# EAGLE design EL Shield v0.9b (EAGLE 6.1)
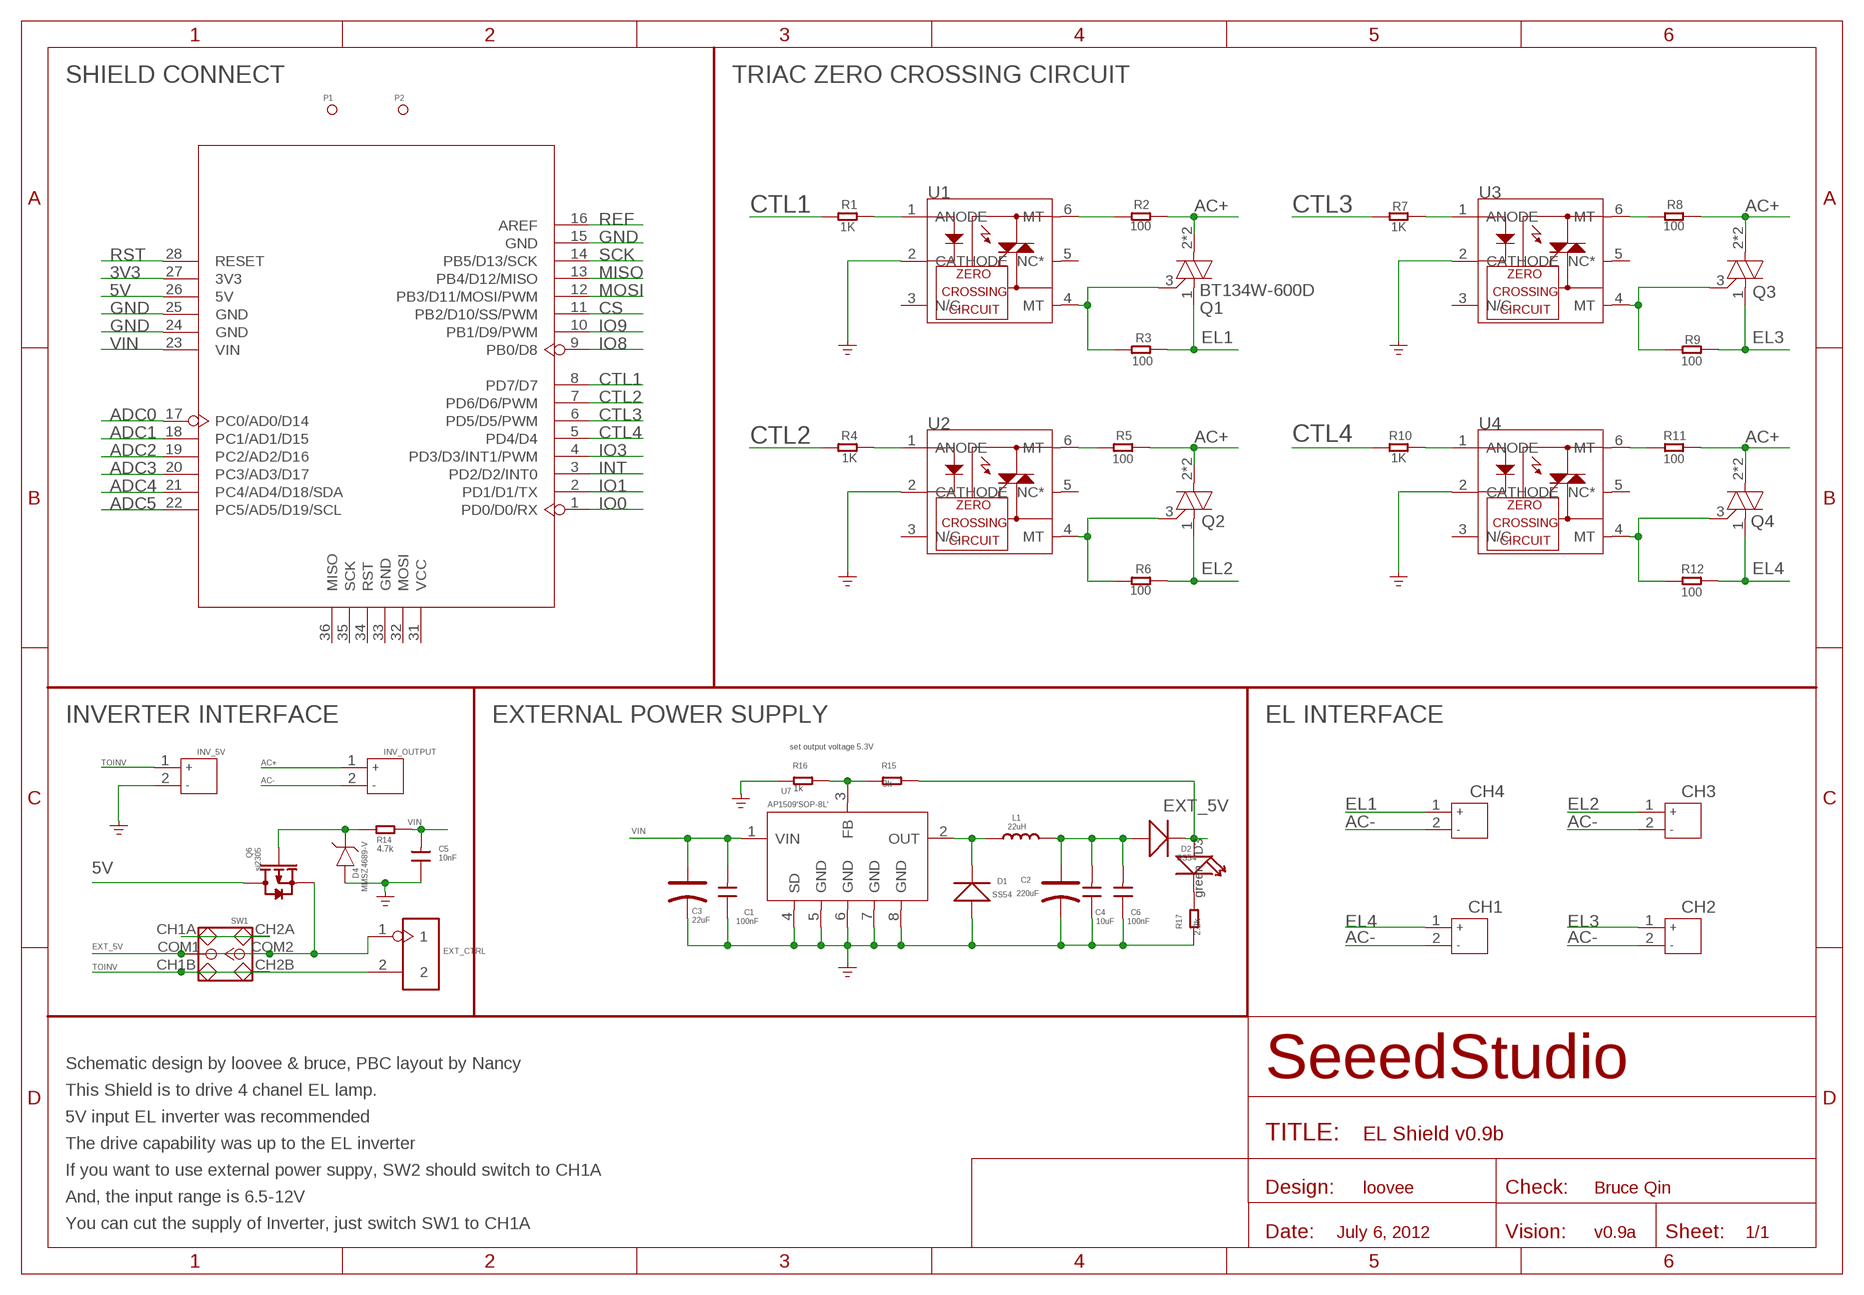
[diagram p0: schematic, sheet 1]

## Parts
C1  100nF  C-0603  [0603]
C2  220uF  CAP-AVX-B  [AVX-B]
C3  22uF  CAP-AVX-A  [AVX-A]
C4  10uF  C-0603  [0603]
C5  10nF  C-0603  [0603]
C6  100nF  C-0603  [0603]
CH1  JACK-JST-2P-PW'SMD'  [JST-SMD-2.0]
CH2  JACK-JST-2P-PW'SMD'  [JST-SMD-2.0]
CH3  JACK-JST-2P-PW'SMD'  [JST-SMD-2.0]
CH4  JACK-JST-2P-PW'SMD'  [JST-SMD-2.0]
D1  SS54  D'MBRS240LT3'  [SMB]
D2  SS54  D'MBRS240LT3'  [SMB]
D3  green  LED'0603'  [LED-0603]
D4  MMSZ4689-V  D-VOL'MMSZ4681'  [SOD123-2.7X1.6]
EXT_CTRL  HEADER-2P-65/35MIL  [2P-2.54-65/35MIL]
INV_5V  JACK-JST-2P-PW'2.0'  [JST-2.0]
INV_OUTPUT  JACK-JST-2P-PW'2.0'  [JST-2.0]
L1  22uH  L'2218'  [2218]
P1  PAD-MARK  [ROUND-MARK-1.0]
P2  PAD-MARK  [ROUND-MARK-1.0]
Q1  BT134W-600D  TRIAC'BT134W-600D'  [SOT-223]
Q2  TRIAC'BT134W-600D'  [SOT-223]
Q3  TRIAC'BT134W-600D'  [SOT-223]
Q4  TRIAC'BT134W-600D'  [SOT-223]
Q6  si2305  MOSFET-P'SI2323CDS/SI2305DS<BR>'  [SOT23]
R1  1K  R-0603  [R0603]
R2  100  R-0805  [R0805]
R3  100  R-0805  [R0805]
R4  1K  R-0603  [R0603]
R5  100  R-0805  [R0805]
R6  100  R-0805  [R0805]
R7  1K  R-0603  [R0603]
R8  100  R-0805  [R0805]
R9  100  R-0805  [R0805]
R10  1K  R-0603  [R0603]
R11  100  R-0805  [R0805]
R12  100  R-0805  [R0805]
R14  4.7k  R-0603  [R0603]
R15  3k  R-0603  [R0603]
R16  1k  R-0603  [R0603]
R17  2.2k  R-0603  [R0603]
SW1  SWITCH-2CH-6P  [6P-2CH-2.54-7.6X3.0]
U1  MOC3063MS  [SM6]
U2  MOC3063MS  [SM6]
U3  MOC3063MS  [SM6]
U4  MOC3063MS  [SM6]
U5  ARDUINO  [ARDUINO]
U7  AP1509'SOP-8L'  [SOP8-6.0-4.9X3.9]

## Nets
3V3: U5.27(3V3)
5V: Q6.3(D) U5.26(5V)
AC+: INV_OUTPUT.1 Q1.2(T2) Q1.TER(T2) Q2.2(T2) Q2.TER(T2) Q3.2(T2) Q3.TER(T2) Q4.2(T2) Q4.TER(T2) R2.2 R5.2 R8.2 R11.2
AC-: CH1.2 CH2.2 CH3.2 CH4.2 INV_OUTPUT.2
ADC0: U5.17(PC0/AD0/D14)
ADC1: U5.18(PC1/AD1/D15)
ADC2: U5.19(PC2/AD2/D16)
ADC3: U5.20(PC3/AD3/D17)
ADC4: U5.21(PC4/AD4/D18/SDA)
ADC5: U5.22(PC5/AD5/D19/SCL)
CS: U5.11(PB2/D10/SS/PWM)
CTL1: R1.2 U5.8(PD7/D7)
CTL2: R4.2 U5.7(PD6/D6/PWM)
CTL3: R7.2 U5.6(PD5/D5/PWM)
CTL4: R10.2 U5.5(PD4/D4)
EL1: CH4.1 Q1.1(T1) R3.2
EL2: CH3.1 Q2.1(T1) R6.2
EL3: CH2.1 Q3.1(T1) R9.2
EL4: CH1.1 Q4.1(T1) R12.2
EXT_5V: D2.- D3.+ EXT_CTRL.1 Q6.2(S) R15.1 SW1.COM1 SW1.COM2
GND: C1.1 C2.- C3.- C4.1 C5.1 C6.1 D1.+ D4.1 INV_5V.2 R16.2 R17.2 U1.2(CATHODE) U2.2(CATHODE) U3.2(CATHODE) U4.2(CATHODE) U5.15(GND) U5.24(GND) U5.25(GND) U7.4(SD) U7.5(GND) U7.6(GND) U7.7(GND) U7.8(GND)
INT: U5.3(PD2/D2/INT0)
IO0: U5.1(PD0/D0/RX)
IO1: U5.2(PD1/D1/TX)
IO3: U5.4(PD3/D3/INT1/PWM)
IO8: U5.9(PB0/D8)
IO9: U5.10(PB1/D9/PWM)
MISO: U5.13(PB4/D12/MISO)
MOSI: U5.12(PB3/D11/MOSI/PWM)
N$1: SW1.CH1A SW1.CH2A
N$2: R4.1 U2.1(ANODE)
N$3: R5.1 U2.6(MT)
N$4: Q2.3(G) R6.1 U2.4(MT)
N$5: R15.2 R16.1 U7.3(FB)
N$6: R7.1 U3.1(ANODE)
N$7: R8.1 U3.6(MT)
N$8: Q3.3(G) R9.1 U3.4(MT)
N$9: D4.2 Q6.1(G) R14.1
N$10: D1.- L1.P$1 U7.2(OUT)
N$11: R1.1 U1.1(ANODE)
N$12: R2.1 U1.6(MT)
N$13: R10.1 U4.1(ANODE)
N$14: Q1.3(G) R3.1 U1.4(MT)
N$15: R11.1 U4.6(MT)
N$16: Q4.3(G) R12.1 U4.4(MT)
N$17: D3.- R17.1
N$18: C2.+ C4.2 C6.2 D2.+ L1.P$2
REF: U5.16(AREF)
RST: U5.28(RESET)
SCK: U5.14(PB5/D13/SCK)
TOINV: EXT_CTRL.2 INV_5V.1 SW1.CH1B SW1.CH2B
VIN: C1.2 C3.+ C5.2 R14.2 U5.23(VIN) U7.1(VIN)
Unconnected: U1.3(N/C) U1.5(NC*) U2.3(N/C) U2.5(NC*) U3.3(N/C) U3.5(NC*) U4.3(N/C) U4.5(NC*) U5.31(VCC) U5.32(MOSI) U5.33(GND) U5.34(RST) U5.35(SCK) U5.36(MISO)

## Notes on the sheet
- SHIELD CONNECT | TRIAC ZERO CROSSING CIRCUIT
- INVERTER INTERFACE | EXTERNAL POWER SUPPLY | EL INTERFACE
- set output voltage 5.3V
- Schematic design by loovee & bruce, PBC layout by Nancy
- This Shield is to drive 4 chanel EL lamp.
- 5V input EL inverter was recommended
- The drive capability was up to the EL inverter
- If you want to use external power suppy, SW2 should switch to CH1A
- loovee | Bruce Qin
- And, the input range is 6.5-12V
- You can cut the supply of Inverter, just switch SW1 to CH1A
- July 6, 2012 | v0.9a

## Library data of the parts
C1 C4-C6 = Discrete:C*: Ceramic Capacitors
C2 C3 = Discrete:CAP*: Electrolytic Capacitors,Tantalum Capacitors and Super Capacitors
CH1-CH4 INV_5V INV_OUTPUT = Connector:JACK-JST-2P-PW
D1 D2 = Discrete:D*
D3 = Discrete:LED*
D4 = template:D-VOL
EXT_CTRL = Connector:HEADER-2P
L1 = Discrete:L*
P1 P2 = Discrete:PAD-MARK; PARTNO: DNP
Q1-Q4 = template:TRIAC: Triac
Q6 = Discrete:MOSFET-P
R1-R12 R14-R17 = Discrete:R*
SW1 = Discrete:SWITCH-2CH-6P
U1-U4 = template:MOC3063*M: 6-Pin DIP Zero-Cross Phototriac Driver Optocoupler(600 Volt Peak)
U5 = moudle:ARDUINO
U7 = IC:AP1509: 150KHz,2A PWM Buck DC/DC Converter

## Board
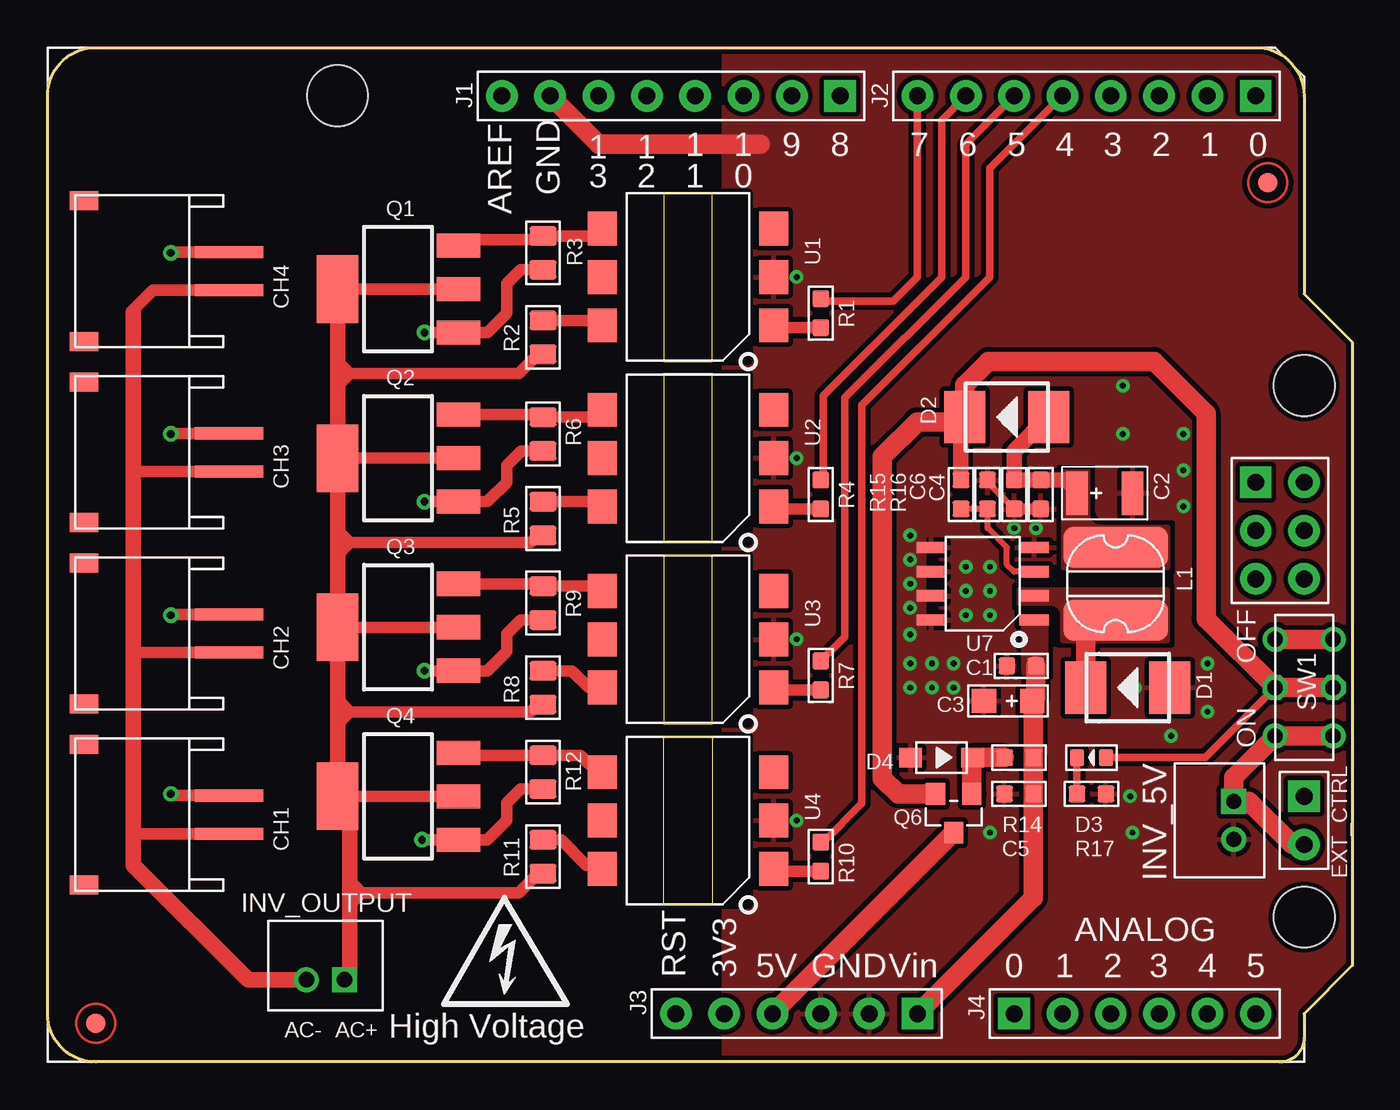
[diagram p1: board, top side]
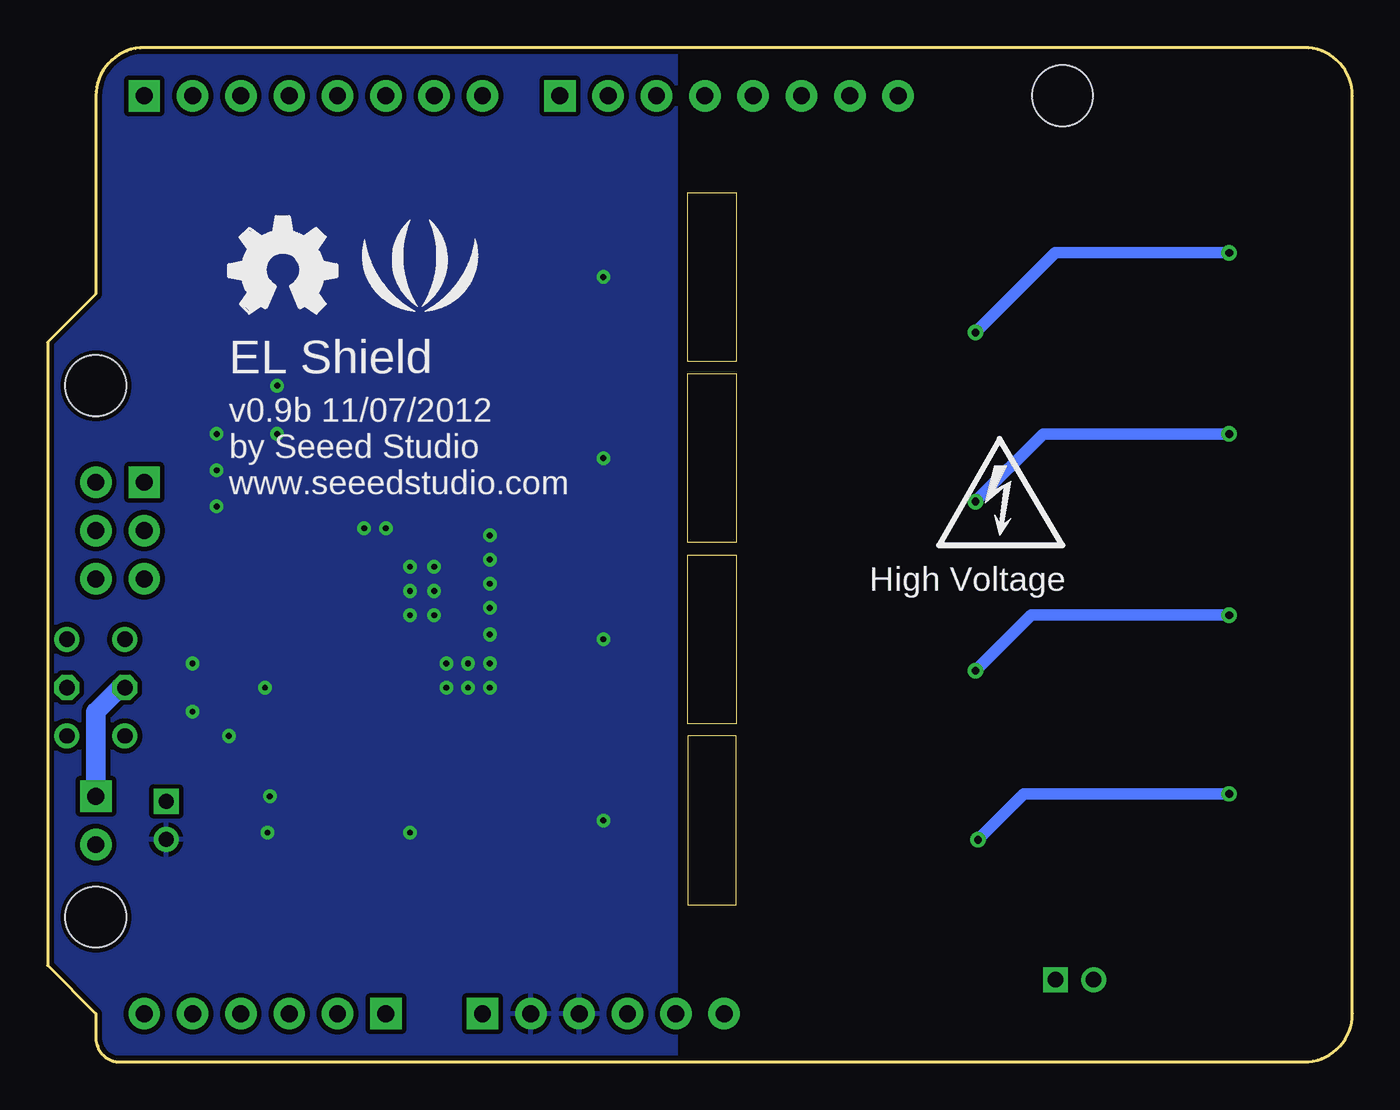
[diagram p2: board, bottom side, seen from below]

Size 68.58 x 53.34 mm. Coordinates in mm from the lower left corner, seen from the top.
Outline: 32.38,17.14 34.92,17.14 34.92,8.25 32.38,8.25 32.38,17.14
Outline: 32.38,17.78 34.92,17.78 34.92,26.67 32.38,26.67 32.38,17.78
Outline: 32.38,27.3 34.92,27.3 34.92,36.19 32.38,36.19 32.38,27.3
Outline: 32.38,36.83 34.92,36.83 34.92,45.72 32.38,45.72 32.38,36.83
Outline: 66.04,2.54 66.04,1.27 arc-90 64.77,0 2.54,0 arc-90 0,2.54 0,50.8 arc-90 2.54,53.34 63.5,53.34 arc-90 66.04,50.8 66.04,40.39 68.58,37.85 68.58,5.08 66.04,2.54
Copper layers (1*16): Top 0.035mm / dielectric 1.5mm / Bottom 0.035mm
Design rules: minimum track width 10mil, minimum drill 12mil, track to track 8mil, track to pad 8mil, pad to pad 8mil, via to via 8mil, smd to smd 0mil, copper to edge 10mil, drill to drill 8mil, minimum pad ring 10mil, minimum via ring 8mil, stop-mask expansion 4mil, vias tented up to drill 100mil, thermal gap 10mil
tRestrict: area 53.2,25.3 to 58.9,25.5; area 46.2,23.7 to 46.6,24; area 46.2,25 to 46.6,25.3; area 46.2,26.3 to 46.6,26.5

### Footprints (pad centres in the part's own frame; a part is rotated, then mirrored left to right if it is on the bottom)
0603 = smd 0.889 x 0.889: 1 -0.762,0; 2 0.762,0
AVX-B = smd 1.143 x 2.286: + -1.46,0; - 1.46,0
AVX-A = smd 1.27 x 1.27: + -1.27,0; - 1.27,0
JST-SMD-2.0 = smd 0.635 x 3.6: 1 -1,5.08; 2 1,5.08 | smd 1 x 1.5: P$1 -3.7,-2.54; P$2 3.7,-2.54
SMB = smd 2.159 x 2.743: + -2.21,0.254; - 2.21,0.254
LED-0603 = smd 0.762 x 0.889: + -0.762,0; - 0.762,0
SOD123-2.7X1.6 = smd 1.2 x 1.02: 1 -1.635,0; 2 1.635,0
2P-2.54-65/35MIL = drill 0.889 pad 1.651 square: 1 0,1.27 | drill 0.889 pad 1.651: 2 0,-1.27
JST-2.0 = drill 0.8 pad 1.3 square: 1 -1,0.75 | drill 0.8 pad 1.3: 2 1,0.75
2218 = smd 2.15 x 5.5: P$1 -1.925,0; P$2 1.925,0
ROUND-MARK-1.0 = smd 1.016 x 1.016: P$1 0,0
SOT-223 = smd 1.27 x 2.286: 1 -2.286,-3.175; 2 0,-3.175; 3 2.286,-3.175 | smd 3.556 x 2.159: TER 0,3.175
SOT23 = smd 1.016 x 1.143: 1 -0.95,-1.016; 2 0.95,-1.016; 3 0,1.016
R0603 = smd 0.889 x 0.889: 1 -0.762,0; 2 0.762,0
R0805 = smd 1.016 x 1.397: 1 -0.889,0; 2 0.889,0
6P-2CH-2.54-7.6X3.0 = drill 0.813 pad 1.27: CH1A -1.524,2.54; CH1B -1.524,-2.54; CH2A 1.524,2.54; CH2B 1.524,-2.54 | drill 0.813 pad 1.27 octagon: COM1 -1.524,0; COM2 1.524,0
SM6 = smd 1.78 x 1.52: 1 -2.54,-4.505; 2 0,-4.505; 3 2.54,-4.505; 4 2.54,4.505; 5 0,4.505; 6 -2.54,4.505
ARDUINO = drill 0.889 pad 1.651 square: 1 63.5,50.8; 9 41.656,50.8; 17 50.8,2.54; 23 45.72,2.54; 36 63.5,30.48 | drill 0.889 pad 1.651: 2 60.96,50.8; 3 58.42,50.8; 4 55.88,50.8; 5 53.34,50.8; 6 50.8,50.8; 7 48.26,50.8; 8 45.72,50.8; 10 39.116,50.8; 11 36.576,50.8; 12 34.036,50.8; 13 31.496,50.8; 14 28.956,50.8; 15 26.416,50.8; 16 23.876,50.8; 18 53.34,2.54; 19 55.88,2.54; 20 58.42,2.54; 21 60.96,2.54; 22 63.5,2.54; 24 43.18,2.54; 25 40.64,2.54; 26 38.1,2.54; 27 35.56,2.54; 28 33.02,2.54; 31 66.04,30.48; 32 66.04,27.94; 33 66.04,25.4; 34 63.5,25.4; 35 63.5,27.94 | hole 3.2: 15.24,50.8; 66.04,35.56; 66.04,7.62
SOP8-6.0-4.9X3.9 = smd 0.6 x 1.55: 1 -1.905,-2.7; 2 -0.635,-2.7; 3 0.635,-2.7; 4 1.905,-2.7; 5 1.905,2.7; 6 0.635,2.7; 7 -0.635,2.7; 8 -1.905,2.7

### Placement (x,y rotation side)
C1  51.18,20.83 0 top
C2  55.56,29.91 0 top
C3  50.48,18.99 180 top
C4  52.2,29.84 90 top
C5  51.05,14.1 0 top
C6  50.8,29.84 90 top
CH1  4.44,13 270 top
CH2  4.44,22.53 270 top
CH3  4.44,32.05 270 top
CH4  4.44,41.58 270 top
D1  56.77,19.94 180 top
D2  50.42,34.16 180 top
D3  54.86,16 180 top
D4  46.99,16 0 top
EXT_CTRL  66.04,12.7 0 top
INV_5V  61.59,12.7 270 top
INV_OUTPUT  14.61,5.08 180 top
L1  56.13,25.15 90 top
P1  2.54,2.03 0 top
P2  64.13,46.23 0 top
Q1  18.41,40.64 90 top
Q2  18.41,31.75 90 top
Q3  18.41,22.86 90 top
Q4  18.41,13.97 90 top
Q6  47.62,13.08 180 top
R1  40.64,39.37 90 top
R2  26.03,38.1 270 top
R3  26.03,42.55 270 top
R4  40.64,29.84 90 top
R5  26.03,28.57 270 top
R6  26.03,33.02 270 top
R7  40.64,20.32 90 top
R8  26.03,19.68 270 top
R9  26.03,24.13 270 top
R10  40.64,10.79 90 top
R11  26.03,10.79 270 top
R12  26.03,15.24 270 top
R14  51.05,16 0 top
R15  48.01,29.84 270 top
R16  49.4,29.84 90 top
R17  54.86,14.1 0 top
SW1  66.04,19.68 0 top
U1  33.65,41.27 90 top
U2  33.65,31.75 90 top
U3  33.65,22.22 90 top
U4  33.65,12.7 90 top
U5  0,0 0 top
U7  49.15,25.15 90 top
U$1  [OSHW_FILLX200_NOTEXT]  59.05,39.37 0 bottom
U$2  [LOGO_SILK]  49.02,41.15 0 bottom

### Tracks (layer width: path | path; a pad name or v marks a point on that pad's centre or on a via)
5V
  Top 1.016: Q6.3 U5.26
AC+
  Top 0.61: 15.88,18.41 15.24,18.41 | Q3.2 Q3.TER | Q4.2 15.88,13.97 Q4.TER | Q2.2 Q2.TER | 15.88,36.19 15.24,36.19 | Q1.2 Q1.TER | 15.88,18.41 15.24,19.05 | 15.88,36.19 15.24,36.83 | 15.88,36.19 15.24,35.56 | R2.2 25.78,37.21 24.77,36.19 15.88,36.19 | R5.2 25.78,27.69 25.4,27.3 15.88,27.3 | 15.88,27.3 15.24,27.3 | R8.2 25.78,18.8 25.4,18.41 15.88,18.41 | R11.2 25.78,9.91 24.77,8.89 16.51,8.89 | 16.51,8.89 15.88,8.89 | 15.88,18.41 15.24,17.78 | 16.51,8.89 15.88,9.52 | 15.88,8.25 16.51,8.89 | 15.88,27.3 15.24,27.94 | 15.88,27.3 15.24,26.67
  Top 0.813: Q4.TER 15.24,17.78 15.24,18.41 15.24,19.05 Q3.TER 15.24,26.67 15.24,27.3 15.24,27.94 Q2.TER 15.24,35.56 15.24,36.19 15.24,36.83 Q1.TER | 15.88,13.97 15.88,9.52 15.88,8.89 15.88,8.25 15.88,4.6 INV_OUTPUT.1
AC-
  Top 0.61: CH4.2 5.52,40.58 4.44,39.5 4.44,39.43 4.51,39.37 4.51,31.05 | CH2.2 4.58,21.53 4.51,21.46 | CH1.2 4.58,12 4.51,11.94 | CH3.2 4.51,31.05 | 4.51,31.05 4.44,30.99
  Top 0.813: 4.51,39.43 4.51,39.37 4.51,21.46 4.51,11.94 4.51,10.35 10.54,4.32 13.59,4.32 INV_OUTPUT.2
CTL1
  Top 0.406: R1.2 40.64,40 44.45,40 45.72,41.27 U5.8
CTL2
  Top 0.406: 40.77,30.61 40.77,35.05 46.99,41.27 46.99,49.53 U5.7
  Top 0.61: R4.2 40.77,30.61
CTL3
  Top 0.406: R7.2 41.91,22.35 41.91,34.92 48.26,41.27 48.26,48.26 U5.6
CTL4
  Top 0.406: R10.2 40.77,11.56 42.8,13.59 42.8,34.54 49.53,41.27 49.53,46.99 U5.5
EL1  (via drill 0.41)
  Top 0.61: R3.2 24.87,41.66 24.13,40.91 24.13,39.37 23.11,38.35 Q1.1 v19.81,38.35 | v6.48,42.55 6.51,42.58 CH4.1
  Bottom 0.61: v19.81,38.35 15.62,42.55 v6.48,42.55
EL2  (via drill 0.41)
  Top 0.61: R6.2 24.89,32.13 24.13,31.37 24.13,30.48 23.11,29.46 Q2.1 v19.81,29.46 | CH3.1 6.51,33.05 v6.48,33.02
  Bottom 0.61: v19.81,29.46 16.26,33.02 v6.48,33.02
EL3  (via drill 0.41)
  Top 0.61: R9.2 24.87,23.24 24.13,22.5 24.13,21.59 23.11,20.57 Q3.1 v19.81,20.57 | v6.48,23.49 6.51,23.53 CH2.1
  Bottom 0.61: v19.81,20.57 16.89,23.49 v6.48,23.49
EL4  (via drill 0.41)
  Top 0.61: R12.2 24.87,14.35 24.13,13.61 24.13,12.7 23.11,11.68 Q4.1 v19.68,11.68 | v6.48,14.1 6.57,14 CH1.1
  Bottom 0.61: v6.48,14.1 17.27,14.1 v19.68,11.68
EXT_5V
  Top 0.406: D3.+ 60.83,16 SW1.COM1
  Top 0.813: R15.1 48.01,33.71 D2.-
  Top 1.016: SW1.COM2 SW1.COM1 60.9,23.3 60.9,34.09 58.16,36.83 49.45,36.83 48.21,35.59 D2.- 47.95,33.66 45.7,33.66 43.88,31.84 43.88,14.92 44.7,14.1 Q6.2
  Bottom 1.016: SW1.COM1 64.77,19.68 66.04,18.41 EXT_CTRL.1
GND  (via drill 0.3 pad 0.64)
  Top 0.305: R16.2 49.4,30.48 C6.1
  Top 0.61: C6.1 C4.1
  Top 1.016: U5.15 28.96,48.26 37.46,48.26
  other vias: 39.37,41.27 39.37,31.75 39.37,22.22 39.37,12.7 51.94,28.07 48.26,23.49 48.26,24.77 48.26,26.03 49.53,26.03 49.53,24.77 49.53,23.49 45.34,23.88 45.34,25.15 45.34,26.42 45.34,27.69 47.62,20.95 47.62,19.68 60.96,20.95 60.96,18.41 56.9,13.97 49.53,12.06 45.34,20.95 45.34,19.68 46.48,20.95 46.48,19.68 59.69,29.21 59.69,31.11 56.52,35.56 56.52,33.02 59.69,33.02 57.02,12.06 59.05,17.14 57.15,19.68 45.34,22.48 50.8,28.07
  pour Bottom: -28.58,53.34 -22.23,53.34 -22.23,50.16 -28.58,50.16
  pour Bottom (isolate 0.254, rank 6): 35.56,53.34 68.58,53.34 68.58,0 35.56,0
  pour Top (isolate 0.254, rank 6): 35.56,53.34 68.58,53.34 68.58,0 35.56,0
  pour Top (no thermals): 45.34,28.32 46.1,28.32 46.1,22.22 45.34,22.22
N$1
  Top 1.016: SW1.CH1A SW1.CH2A
N$2
  Top 0.61: R4.1 38.29,29.08 U2.1
N$3
  Top 0.61: R5.1 28.9,29.46 U2.6
N$4
  Top 0.61: Q2.3 25.91,34.04 R6.1 28.77,33.91 U2.4
N$5
  Top 0.305: U7.3 50.8,25.78 50.42,26.16 50.42,27.05 49.4,28.07 R16.1 R15.2
N$6
  Top 0.61: R7.1 38.29,19.56 U3.1
N$7
  Top 0.61: R8.1 27.56,20.57 28.45,19.68 U3.6
N$8
  Top 0.61: Q3.3 25.91,25.15 R9.1 28.9,25.02 U3.4
N$9
  Top 1.016: Q6.1 48.57,16 48.58,16 D4.2 R14.1
N$10
  Top 1.016: D1.- 54.56,22.94 54.84,23.22 L1.P$1
  pour Top (isolate 0.254, no thermals): 51.05,24.83 51.05,24.13 52.7,24.13 arc-90 53.34,23.49 53.34,22.16 58.86,22.16 58.86,24.83
N$11
  Top 0.61: R1.1 38.29,38.61 U1.1
N$12
  Top 0.61: R2.1 28.89,38.99 U1.6 | U1.6 29.08,38.73 | 29.21,38.73 U1.6
N$13
  Top 0.61: R10.1 38.29,10.03 U4.1
N$14
  Top 0.61: Q1.3 21.97,42.93 22.29,43.24 25.84,43.24 R3.1 28.77,43.43 U1.4
N$15
  Top 0.61: R11.1 26.99,11.68 28.32,10.35 28.96,10.35 U4.6
N$16
  Top 0.61: Q4.3 21.72,16.13 R12.1 28,16.13 28.89,15.24 U4.4
N$17
  Top 0.406: D3.- R17.1
N$18
  Top 0.61: 53.4,30.61 C2.+
  Top 0.813: 53.97,30.04 C2.+ | 53.4,30.61 C4.2 C6.2 50.8,32.13 52.58,33.91 D2.+
  pour Top (isolate 0.254, no thermals): 54.67,31.05 54.67,28.77 arc90 55.31,28.13 58.86,28.13 58.86,25.97 53.4,25.97 53.4,31.05
TOINV
  Top 1.016: SW1.CH2B SW1.CH1B 62.34,14.97 INV_5V.1 63.13,13.7 65.41,11.43 EXT_CTRL.2
VIN
  Top 1.016: C1.2 51.94,19.18 C3.+ 51.82,18.92 R14.2 C5.2 51.82,8.64 U5.23
  pour Top (isolate 0.254, no thermals): 52.45,23.37 52.45,20.45 51.31,20.45 51.31,23.37

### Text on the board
tPlace: J1 | J2 | OFF | ON | J3 | J4 | AC- | AC+ | High Voltage
bPlace: EL Shield | v0.9b 11/07/2012 | by Seeed Studio | www.seeedstudio.com | High Voltage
